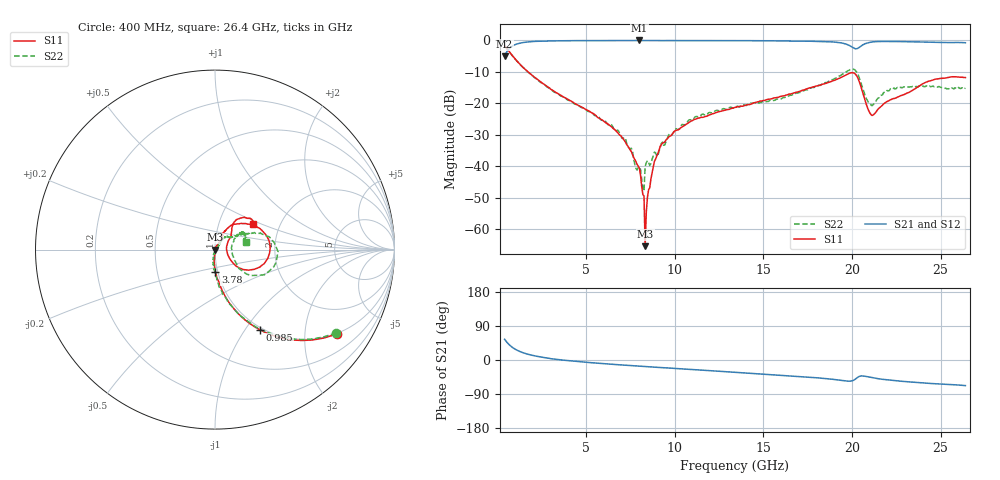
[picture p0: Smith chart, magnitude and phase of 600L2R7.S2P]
!  American Technical Ceramics  Date:  10/27/06
!  One Norden Lane
!  Huntington Station,  NY.  11746-2102
!  Tel:  (631) 622-4700  Fax:  (631) 622-4748
!  Part Number  600L2R7
!  Description: Ultra Low ESR Microwave capacitors
!  Application: Coupling, Bypass, Tuning, DC Block
!  Filters, Matching
# GHZ S DB R 50
! Freq  |S11|  S11 Ph  |S21|  S21 Ph  |S12|  S12 Ph  |S22|  S22 Ph
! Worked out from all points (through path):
!   401 points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, 400 MHz to 26.4 GHz, reference 50 ohm
!   highest |S21| = 0.00 dB at 8.005 GHz (marker M1); lowest = -5.1 dB at 400 MHz (marker M2)
!   group delay of S21, straight-line fit = 8.93 ps
!   lowest |S11| = -65.4 dB at 8.33 GHz (marker M3), VSWR 1.00, Z = 50.1 + j0.0015 ohm
!   |S11| at or under -10 dB: 1.726 GHz to end of sweep
!   |S22| runs from -47.9 to -1.7 dB; largest |S21 - S12| = 0.015
!   S11 on the Smith chart (normalised r, x): 400 MHz: 0.98, -2.89; 985 MHz: 0.97, -1.17; 3.78 GHz: 0.97, -0.25; 26.4 GHz: 1.46, +0.45
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0.4  -1.67 -34.8  -5.06 54.7  -5.10 54.6  -1.73 -34.5
0.985  -5.83 -60.8  -1.35 28.8  -1.39 28.9  -5.87 -60.6
1.895  -10.81 -76.3  -0.38 13.1  -0.42 13.2  -10.89 -76.7
3.78  -18.13 -89.0  -0.09 -0.7  -0.12 -0.5  -18.07 -90.9
4.755  -21.19 -91.5  -0.05 -5.0  -0.07 -4.8  -21.38 -97.0
6.835  -29.73 -92.4  -0.03 -12.6  -0.01 -12.2  -28.84 -101.5
8.005  -40.64 -68.5  0.00 -16.3  -0.01 -16.0  -40.31 -61.0
8.135  -46.43 -70.7  -0.02 -16.9  -0.01 -16.5  -44.02 -40.4
8.2  -48.99 -51.2  -0.03 -17.0  -0.01 -16.7  -46.77 -47.2
8.33  -65.42 1.6  -0.04 -17.4  -0.01 -17.0  -40.06 -42.4
8.46  -49.78 60.4  -0.04 -17.8  -0.01 -17.4  -38.23 -8.5
8.785  -40.36 71.3  -0.04 -18.6  -0.01 -18.3  -36.69 6.9
9.11  -35.03 70.3  -0.04 -19.7  -0.01 -19.4  -35.29 30.5
10.865  -25.83 59.7  -0.03 -24.9  -0.01 -24.8  -25.20 57.3
13.4  -21.30 61.9  -0.04 -32.5  -0.01 -32.5  -21.05 50.8
17.755  -14.85 51.8  -0.26 -46.0  -0.21 -46.4  -14.93 29.2
20.03  -10.25 1.3  -2.20 -54.6  -2.16 -55.2  -9.16 -6.2
20.42  -13.21 -31.6  -2.18 -43.1  -2.13 -43.7  -12.06 -35.3
21.07  -23.57 -6.2  -0.54 -45.7  -0.50 -46.3  -20.42 -2.1
22.11  -19.05 38.9  -0.33 -52.9  -0.29 -53.6  -15.93 32.3
24.45  -12.80 50.2  -0.56 -62.0  -0.52 -62.8  -14.72 26.5
26.4  -11.81 34.0  -0.73 -67.5  -0.70 -68.4  -15.10 14.6
